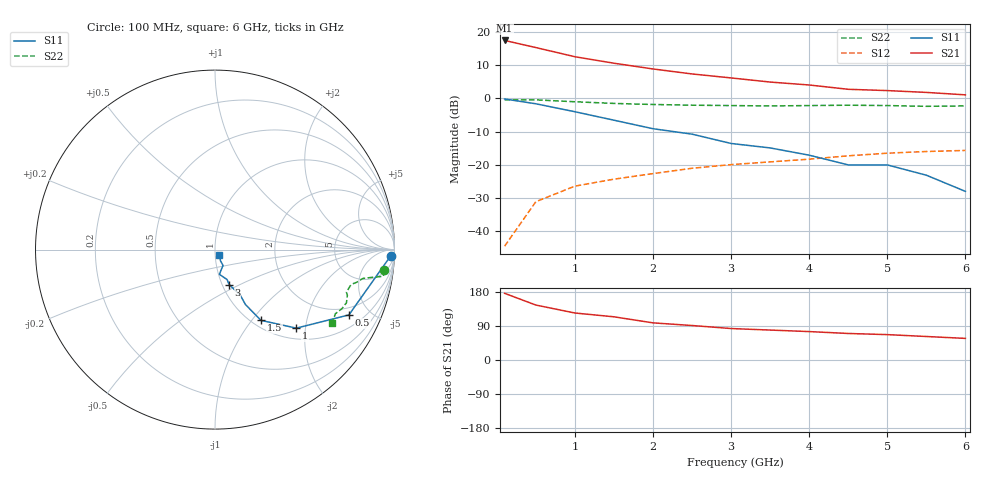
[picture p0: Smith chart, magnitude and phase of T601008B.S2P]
!AT-60100
!S-PARAMETERS at Vce=8V  Ic=3mA.  LAST UPDATED 07-21-92
# ghz s ma r 50
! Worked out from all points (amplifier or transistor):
!   13 points, 100 MHz to 6 GHz, reference 50 ohm
!   highest |S21| = 17.4 dB at 100 MHz (marker M1)
!   |S21| within 3 dB of that: start of sweep to 656.7 MHz
!   unconditionally stable (mu >= 1): 2.096 GHz to end of sweep
!   at 1 GHz: K = 0.62, MSG = 19.5 dB, |S12| = -26.4 dB
!   at 3 GHz: K = 1.11, MAG = 11.0 dB, |S12| = -19.9 dB
!   at 6 GHz: K = 1.21, MAG = 5.6 dB, |S12| = -15.7 dB
!   S11 on the Smith chart (normalised r, x): 100 MHz: 25, -43; 500 MHz: 1.58, -3.70; 1 GHz: 1.23, -1.78; 1.5 GHz: 1.10, -1.11; 3 GHz: 1.08, -0.44; 6 GHz: 1.05, -0.07
0.1  0.98 -2.0  7.43 176.0  0.006 83.0  0.95 -7.0
0.5  0.83 -26.0  5.81 145.0  0.028 78.0  0.95 -9.0
1  0.63 -44.0  4.23 124.0  0.048 70.0  0.89 -10.0
1.5  0.47 -57.0  3.38 114.0  0.061 68.0  0.84 -11.0
2  0.35 -61.0  2.77 98.0  0.074 67.0  0.81 -13.0
2.5  0.29 -61.0  2.33 91.0  0.089 69.0  0.79 -14.0
3  0.21 -68.0  2.03 83.0  0.101 69.0  0.78 -15.0
3.5  0.18 -68.0  1.76 79.0  0.111 70.0  0.77 -18.0
4  0.14 -80.0  1.59 75.0  0.122 73.0  0.78 -19.0
4.5  0.1 -64.0  1.37 70.0  0.137 71.0  0.79 -22.0
5  0.1 -63.0  1.31 67.0  0.15 71.0  0.78 -25.0
5.5  0.07 -64.0  1.23 62.0  0.159 69.0  0.76 -28.0
6  0.04 -53.0  1.13 57.0  0.165 67.0  0.77 -32.0
